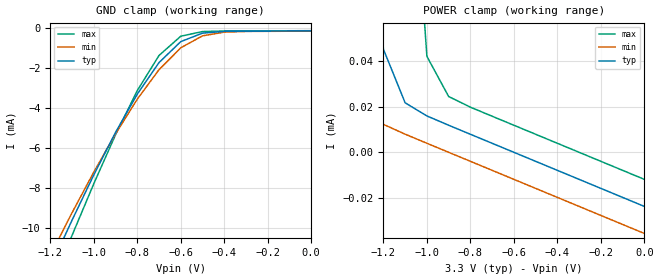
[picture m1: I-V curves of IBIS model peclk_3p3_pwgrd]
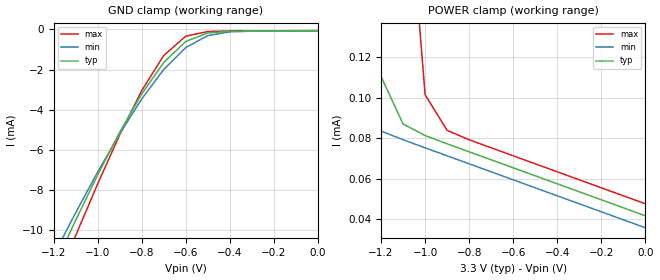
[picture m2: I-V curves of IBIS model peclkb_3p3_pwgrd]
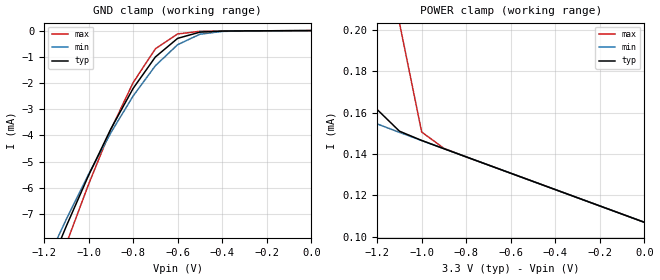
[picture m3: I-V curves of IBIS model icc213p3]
[IBIS ver]   2.1
[File name]   mpc9600.ibs
[File Rev]   2.2   {date modifine 4/29/2002}
[Date]   January 9th, 2002
[Disclaimer]   This information is for modeling purposes only
|   and is not guaranteed.
[Source]   Timing Solutions Operations
[Copyright]   Copyright 2001, Motorola Incorporated,
|   all rights reserved.
| Component MPC9600 for 3.3V Application!
[Component]   MPC96003p3
[Manufacturer]   Motorola
[Package]
|   typ   min   max
R_pkg   0.048   .038   0.053
L_pkg   6.045nH   5.084nH   7.950nH
C_pkg   0.813pF   0.560pF   1.157pF
[Pin]   signal_name model_name R_pin L_pin   C_pin
2   CCLK   icc043p3   0.04   0.35nH   0.053pF
3   PCLK   peclk_3p3_pwgrd   0.04   0.35nH   0.053pF
4   PCLK_BAR   peclkb_3p3_pwgrd  0.04   0.35nH   0.053pF
6   REF_SEL   icc023p3   0.04   0.35nH   0.053pF
7   FSEL_FB   icc023p3   0.04   0.35nH   0.053pF
9   FSELA   icc023p3   0.04   0.35nH   0.053pF
10   FSELB   icc023p3   0.04   0.35nH   0.053pF
11   FSELC   icc023p3   0.04   0.35nH   0.053pF
14   OEB   icc043p3   0.04   0.35nH   0.053pF
15   QC6   occ013p3   0.04   0.35nH   0.053pF
16   QC5   occ013p3   0.04   0.35nH   0.053pF
18   QC4   occ013p3   0.04   0.35nH   0.053pF
19   QC3   occ013p3   0.04   0.35nH   0.053pF
21   QC2   occ013p3   0.04   0.35nH   0.053pF
22   QC1   occ013p3   0.04   0.35nH   0.053pF
23   QC0   occ013p3   0.04   0.35nH   0.053pF
26   QB6   occ013p3   0.04   0.35nH   0.053pF
27   QB5   occ013p3   0.04   0.35nH   0.053pF
28   QB4   occ013p3   0.04   0.35nH   0.053pF
30   QB3   occ013p3   0.04   0.35nH   0.053pF
31   QB2   occ013p3   0.04   0.35nH   0.053pF
33   QB1   occ013p3   0.04   0.35nH   0.053pF
34   QB0   occ013p3   0.04   0.35nH   0.053pF
35   QFB   occ013p3   0.04   0.35nH   0.053pF
38   QA6   occ013p3   0.04   0.35nH   0.053pF
39   QA5   occ013p3   0.04   0.35nH   0.053pF
40   QA4   occ013p3   0.04   0.35nH   0.053pF
42   QA3   occ013p3   0.04   0.35nH   0.053pF
43   QA2   occ013p3   0.04   0.35nH   0.053pF
45   QA1   occ013p3   0.04   0.35nH   0.053pF
46   QA0   occ013p3   0.04   0.35nH   0.053pF
47   FB_IN   icc213p3   0.04   0.35nH   0.053pF
|Component Inputs and Outputs at 2.5V Application
[Component]   MPC96002p5
[Manufacturer]   Motorola
[Package]
|   typ   min   max
R_pkg   0.048   .038   0.053
L_pkg   6.045nH   5.084nH   7.950nH
C_pkg   0.813pF   0.560pF   1.157pF
[Pin]   signal_name model_name R_pin L_pin   C_pin
2   CCLK   icc022p5   0.04   0.35nH   0.053pF
3   PCLK   peclk_2p5_pwgrd   0.04   0.35nH   0.053pF
4   PCLKB   peclkb_2p5_pwgrd   0.04   0.35nH   0.053pF
6   REF_SEL   icc022p5   0.04   0.35nH   0.053pF
7   FSEL_FB   icc022p5   0.04   0.35nH   0.053pF
9   FSELA   icc022p5   0.04   0.35nH   0.053pF
10   FSELB   icc022p5   0.04   0.35nH   0.053pF
11   FSELC   icc022p5   0.04   0.35nH   0.053pF
14   OEB   icc042p5   0.04   0.35nH   0.053pF
15   QC6   occ012p5   0.04   0.35nH   0.053pF
16   QC5   occ012p5   0.04   0.35nH   0.053pF
18   QC4   occ012p5   0.04   0.35nH   0.053pF
19   QC3   occ012p5   0.04   0.35nH   0.053pF
21   QC2   occ012p5   0.04   0.35nH   0.053pF
22   QC1   occ012p5   0.04   0.35nH   0.053pF
23   QC0   occ012p5   0.04   0.35nH   0.053pF
26   QB6   occ012p5   0.04   0.35nH   0.053pF
27   QB5   occ012p5   0.04   0.35nH   0.053pF
28   QB4   occ012p5   0.04   0.35nH   0.053pF
30   QB3   occ012p5   0.04   0.35nH   0.053pF
31   QB2   occ012p5   0.04   0.35nH   0.053pF
33   QB1   occ012p5   0.04   0.35nH   0.053pF
34   QB0   occ012p5   0.04   0.35nH   0.053pF
35   QFB   occ012p5   0.04   0.35nH   0.053pF
38   QA6   occ012p5   0.04   0.35nH   0.053pF
39   QA5   occ012p5   0.04   0.35nH   0.053pF
40   QA4   occ012p5   0.04   0.35nH   0.053pF
42   QA3   occ012p5   0.04   0.35nH   0.053pF
43   QA2   occ012p5   0.04   0.35nH   0.053pF
45   QA1   occ012p5   0.04   0.35nH   0.053pF
46   QA0   occ012p5   0.04   0.35nH   0.053pF
47   FB_IN   icc212p5   0.04   0.35nH   0.053pF
| Models and submodels in the file (12): peclk_3p3_pwgrd (Input), peclkb_3p3_pwgrd (Input), icc213p3 (Input), icc023p3 (Input), icc043p3 (Input), occ013p3 (Output), peclk_2p5_pwgrd (Input), peclkb_2p5_pwgrd (Input), icc212p5 (Input), icc042p5 (Input), icc022p5 (Input), occ012p5 (Output)
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|This is a Model of a PECL Input with a 25,000 ohm Pull_down at 3.3V
[Model]   peclk_3p3_pwgrd
Model_type   Input
Vmeas=1.5
Vinl=0.8
Vinh=2.0
| Variable   typ   min   max
C_comp   5p   5p   5p
[Temperature Range]   27.00   100.00   -45.00
[Power Clamp Reference]   3.30V   3.00V   3.60V
[Gnd Clamp Reference]   0.000V   0.000V   0.000V
[Voltage Range]   3.30V   3.00V   3.60V
[Pulldown Reference]   0.000V   0.000V   0.000V
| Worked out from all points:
|   GND clamp passes 1 mA (typ) near -0.63 V on its own axis
|   POWER clamp passes 1 mA (typ) near -1.46 V on its own axis
[GND_clamp]
| voltage   I(typ)   I(min)   I(max)
-3.3V     -65.58mA   -61.83mA   -70.36mA
-1.2V     -11.96mA   -11.35mA   -13.02mA
-1.1V     -9.594mA   -9.224mA   -10.36mA
-1V       -7.329mA   -7.188mA   -7.771mA
-900mV    -5.205mA   -5.279mA   -5.323mA
-800mV    -3.291mA   -3.546mA   -3.115mA
-700mV    -1.714mA   -2.069mA   -1.359mA
-600mV    -666.8uA   -975.9uA   -396.7uA
-500mV    -241.6uA   -377.6uA   -163.2uA
-400mV    -155.7uA   -192.2uA   -135.8uA
1.97fV    -130.7uA   -142.6uA   -118.8uA
[POWER_clamp]
| voltage   I(typ)  I(min)  I(max)
-3.3V     27.08mA    21.42mA    33.95mA
-1.5V     1.27mA     194.8uA    3.742mA
-1.4V     587.9uA    51.94uA    2.515mA
-1.3V     181.2uA    19.57uA    1.462mA
-1.2V     45.26uA    12.26uA    649.8uA
-1.1V     21.73uA    7.958uA    178.7uA
-1V       15.97uA    3.969uA    42.13uA
-900mV    11.89uA    5.703nA    24.5uA
-800mV    7.921uA    -3.955uA   19.82uA
1.97fV    -23.76uA   -35.64uA   -11.88uA
|This is a Model of a PECL_BAR Input with a 25,000 ohm Pull_Up at 3.3V
[Model]   peclkb_3p3_pwgrd
Model_type   Input
Vmeas=1.5
Vinl=.8
Vinh=2.0
| Variable   typ   min   max
C_comp   5p   5p   5p
[Temperature Range]   27.00   100.00   -45.00
[Power Clamp Reference]   3.30V   3.00V   3.60V
[Gnd Clamp Reference]   0.000V   0.000V   0.000V
[Voltage Range]   3.30V   3.00V   3.60V
[Pulldown Reference]   0.000V   0.000V   0.000V
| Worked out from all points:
|   GND clamp passes 1 mA (typ) near -0.64 V on its own axis
|   POWER clamp passes 1 mA (typ) near -1.45 V on its own axis
[GND_clamp]
| voltage   I(typ)   I(min)   I(max)
-3.3V     -65.51mA   -61.76mA   -70.3mA
-1.2V     -11.89mA   -11.28mA   -12.96mA
-1.1V     -9.53mA    -9.154mA   -10.3mA
-1V       -7.265mA   -7.118mA   -7.713mA
-900mV    -5.141mA   -5.209mA   -5.265mA
-800mV    -3.227mA   -3.475mA   -3.057mA
-700mV    -1.649mA   -1.999mA   -1.301mA
-600mV    -601.9uA   -905.3uA   -337.6uA
-500mV    -176.4uA   -306.5uA   -103.9uA
-400mV    -90.4uA    -121uA     -76.41uA
1.97fV    -65.34uA   -71.29uA   -59.4uA
[POWER_clamp]
| voltage   I(typ)  I(min)  I(max)
-3.3V     27.15mA    21.49mA    34.01mA
-1.5V     1.335mA    265.9uA    3.8mA
-1.4V     652.9uA    123.2uA    2.573mA
-1.3V     246.4uA    90.85uA    1.52mA
-1.2V     110.6uA    83.55uA    708.8uA
-1.1V     87.07uA    79.24uA    237.9uA
-1V       81.31uA    75.25uA    101.5uA
-900mV    77.23uA    71.29uA    83.9uA
-800mV    73.26uA    67.33uA    79.23uA
1.97fV    41.58uA    35.65uA    47.52uA
|This is a Model of an CMOS Input with a 25,000 ohm Pull_down at 3.3V
[Model]   icc213p3
Model_type   Input
Vmeas=1.5
Vinl=.8
Vinh=2.0
| Variable   typ   min   max
C_comp   5p   5p   5p
[Temperature Range]   27.00   100.00   -45.00
[Power Clamp Reference]   3.30V   3.00V   3.60V
[Gnd Clamp Reference]   0.000V   0.000V   0.000V
[Voltage Range]   3.30V   3.00V   3.60V
[Pulldown Reference]   0.000V   0.000V   0.000V
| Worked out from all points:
|   GND clamp passes 1 mA (typ) near -0.70 V on its own axis
|   POWER clamp passes 1 mA (typ) near -1.52 V on its own axis
[GND_clamp]
| voltage   I(typ)   I(min)   I(max)
-3.3V     -59.4mA    -55.11mA   -65.17mA
-1.2V     -9.523mA   -9.03mA    -10.54mA
-1.1V     -7.468mA   -7.206mA   -8.143mA
-1V       -5.53mA    -5.487mA   -5.871mA
-900mV    -3.755mA   -3.903mA   -3.783mA
-800mV    -2.21mA    -2.498mA   -1.989mA
-700mV    -1.008mA   -1.343mA   -696.5uA
-600mV    -296.7uA   -538.1uA   -129.1uA
-500mV    -59.69uA   -139.6uA   -27.92uA
-400mV    -19.24uA   -31.94uA   -16.12uA
1.97fV    -4.613pA   -430.8pA   -3pA
[POWER_clamp]
| voltage   I(typ)  I(min)  I(max)
-3.3V     21.01mA    16.19mA    27.41mA
-1.5V     858.9uA    250.7uA    2.546mA
-1.4V     435.3uA    177.5uA    1.67mA
-1.3V     219.2uA    159.8uA    954uA
-1.2V     161.6uA    154.6uA    447.4uA
-1.1V     151.1uA    150.5uA    203.6uA
-1V       146.6uA    146.5uA    150.6uA
-900mV    142.6uA    142.6uA    142.8uA
1.97fV    106.9uA    106.9uA    106.9uA
